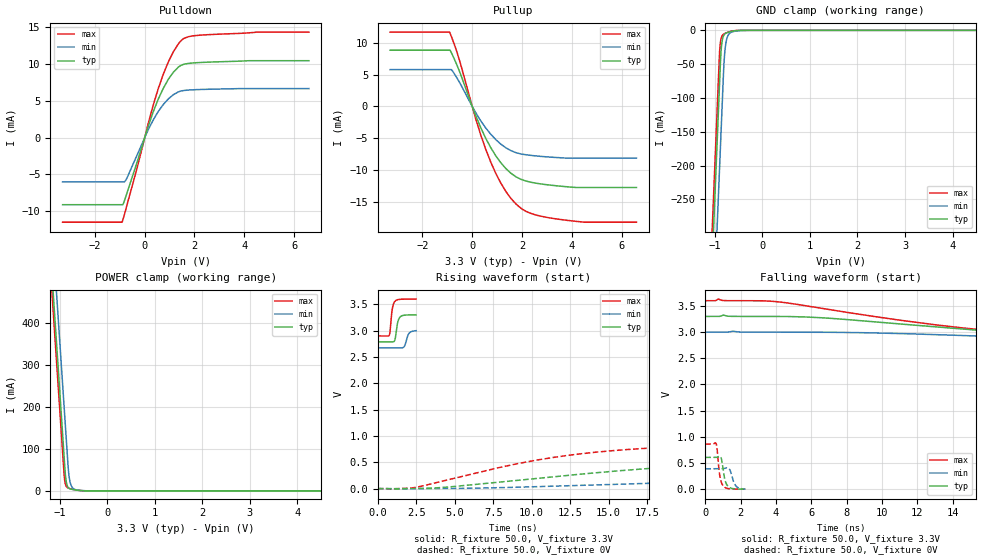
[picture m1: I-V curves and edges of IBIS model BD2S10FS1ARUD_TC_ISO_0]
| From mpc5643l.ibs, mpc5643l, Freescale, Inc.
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| *** New cell (Generated with 5.14beta1 (Sep 20 2010 13:23:23))
[Model]   BD2S10FS1ARUD_TC_ISO_0
Model_type I/O
Polarity   Non-Inverting
Enable   Active-Low
| CAP_THRESHOLD on pad pad is "CMOS" :
| Rising=10.0% of VDDE1   Falling=90.0% of VDDE1
| C_comp min and max val. don't necessarily correlate with the min and max pvt
| but are the smallest and greatest pad capacitance found.
| var   typ   min   max
C_comp   2.15700pF  2.04013pF  2.29327pF
Vinl = 1.05V | Dummy value overriden by next lines
Vinh = 2.34V | Dummy value overriden by next lines
Vmeas = 1.65V   | Reference voltage for timing measurements
Cref  = 25.0pF   | Timing specification test load capacitance value
Rref  = 1.0MOhm   | Timing specification test load resistance value
Vref  = 1.65V   | Timing specification test load voltage
[Model Spec]
| TIME_THRESHOLD on pin ipp_ind is "CORE" :
| Rising=40.0% of VDD   Falling=60.0% of VDD
Vinl 1.32350V 1.20950V 1.42250V
Vinh 1.90350V 1.72650V 2.05550V
| variable   typ   min   max
[Temperature Range] 25.0 150.0 -40.0
| variable   typ   min   max
[Voltage Range] 3.3V 3.0V 3.6V
| variable   typ   min   max
[POWER Clamp Reference] 3.3V 3.0V 3.6V
| variable   typ   min   max
[GND Clamp Reference] 0V 0V 0V
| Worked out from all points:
|   slope of the pulldown table from 0 to 0.495 V, typ, clamps not added: 103 ohm
|   slope of the pullup table from 0 to 0.495 V, typ, clamps not added: 108 ohm
|   GND clamp passes 1 mA (typ) near -0.61 V on its own axis
|   POWER clamp passes 1 mA (typ) near -0.57 V on its own axis
|   rising waveform, R_fixture 50.0, V_fixture 3.3V: 20-80 % time 176ps typ, 215ps min, 157ps max; typ from 2.79 V to 3.3 V
|   falling waveform, R_fixture 50.0, V_fixture 3.3V: 20-80 % time 12.8ns typ, 19.9ns min, 9.33ns max; typ from 3.3 V to 2.79 V
|   rising waveform, R_fixture 50.0, V_fixture 0V: 20-80 % time 16ns typ, 31.9ns min, 9.41ns max; typ from 0 V to 0.606 V
|   falling waveform, R_fixture 50.0, V_fixture 0V: 20-80 % time 202ps typ, 238ps min, 181ps max; typ from 0.606 V to 0 V
[POWER Clamp]
-3.3V     4.147A     4.265A     4.103A
-1.21V    593.6mA    712.4mA    550.2mA
-1.14V    474.6mA    593.4mA    431.2mA
-1.07V    355.6mA    474.4mA    312.2mA
-1V       236.6mA    355.4mA    193.2mA
-900mV    66.63mA    185.4mA    27.75mA
-870mV    26.01mA    134.4mA    12.15mA
-820mV    7.991mA    51.43mA    6.71mA
-790mV    5.39mA     24.66mA    5.573mA
-740mV    3.621mA    8.522mA    4.182mA
-500mV    402.7uA    702.3uA    321.1uA
6.6V      0A         0A         0A
[GND Clamp]
-3.3V     -4.158A    -4.283A    -4.111A
-1.08V    -384.3mA   -509.2mA   -336.5mA
-910mV    -95.27mA   -220.2mA   -47.53mA
-890mV    -61.27mA   -186.2mA   -22.28mA
-880mV    -44.27mA   -169.2mA   -16.28mA
-860mV    -23.44mA   -135.2mA   -10.07mA
-810mV    -7.304mA   -52.22mA   -5.488mA
-790mV    -5.469mA   -31.98mA   -4.717mA
-760mV    -3.985mA   -16.09mA   -3.79mA
-680mV    -2.058mA   -3.959mA   -1.879mA
-460mV    -100.3uA   -366.4uA   -40.84uA
6.6V      10.86nA    3.471uA    69.11pA
| variable   typ   min   max
[Pullup Reference] 3.3V 3.0V 3.6V
| variable   typ   min   max
[Pulldown Reference] 0V 0V 0V
[Pullup]
-3.3V     8.828mA    5.778mA    11.67mA
-910mV    8.828mA    5.778mA    11.67mA
-830mV    8.358mA    5.778mA    10.89mA
-530mV    5.681mA    3.906mA    7.464mA
340mV     -3.31mA    -2.242mA   -4.446mA
740mV     -6.438mA   -4.34mA    -8.697mA
950mV     -7.768mA   -5.218mA   -10.53mA
1.35V     -9.742mA   -6.484mA   -13.33mA
1.96V     -11.44mA   -7.454mA   -15.99mA
2.57V     -12.05mA   -7.77mA    -17.05mA
3.78V     -12.6mA    -8.107mA   -17.86mA
6.6V      -12.72mA   -8.115mA   -18.17mA
[Pulldown]
-3.3V     -9.096mA   -6.007mA   -11.47mA
-910mV    -9.096mA   -6.007mA   -11.47mA
-860mV    -8.955mA   -6.007mA   -10.95mA
-730mV    -7.701mA   -5.58mA    -9.361mA
-270mV    -2.95mA    -2.093mA   -3.641mA
140mV     1.518mA    1.051mA    1.902mA
540mV     5.179mA    3.516mA    6.592mA
950mV     7.904mA    5.249mA    10.26mA
1.15V     8.857mA    5.814mA    11.62mA
1.53V     9.89mA     6.36mA     13.34mA
2.57V     10.23mA    6.552mA    13.95mA
6.6V      10.42mA    6.642mA    14.3mA
[Ramp]
dV/dt_r 363.82411mV/16.01548ns 233.53819mV/31.8706ns 516.40158mV/9.40995ns
dV/dt_f 307.73137mV/12.83706ns 196.81296mV/19.89569ns 420.29549mV/9.33353ns
R_load = 50.0
| Removed startup time: 0s 0s 0s  .
| Removed end time: 2.485ns.
[Rising Waveform]
R_fixture   = 50.0
V_fixture   = 3.3V
V_fixture_min = 3.0V
V_fixture_max = 3.6V
0s        2.787V     2.672V     2.9V
748ps     2.787V     2.672V     2.915V
801ps     2.787V     2.672V     2.995V
939ps     2.785V     2.672V     3.409V
1.112ns   2.825V     2.672V     3.556V
1.284ns   3.145V     2.672V     3.587V
1.426ns   3.251V     2.671V     3.594V
1.727ns   3.293V     2.701V     3.598V
2.048ns   3.298V     2.955V     3.599V
2.487ns   3.3V       3V         3.6V
| Removed startup time: 0s 0s 0s  .
| Removed end time: 89.5ns.
[Falling Waveform]
R_fixture   = 50.0
V_fixture   = 3.3V
V_fixture_min = 3.0V
V_fixture_max = 3.6V
0s        3.3V       3V         3.6V
750ps     3.299V     3V         3.631V
4.1ns     3.3V       3V         3.579V
7ns       3.266V     2.997V     3.431V
14.65ns   3.057V     2.934V     3.078V
17.75ns   2.98V      2.898V     2.991V
21.4ns    2.905V     2.856V     2.948V
28.2ns    2.837V     2.783V     2.92V
40.4ns    2.803V     2.715V     2.905V
89.6ns    2.787V     2.672V     2.9V
| Removed startup time: 0s 0s 0s  .
| Removed end time: 113.2ns.
[Rising Waveform]
R_fixture   = 50.0
V_fixture   = 0V
V_fixture_min = 0V
V_fixture_max = 0V
0s        18.72nV    2.005uV    15.84nV
900ps     324.5uV    1.89uV     -10.23mV
2.5ns     1.08mV     -197.2uV   26.1mV
8.8ns     148.8mV    24.33mV    457.2mV
12.65ns   260.5mV    56.06mV    642.3mV
16.8ns    364.8mV    93.16mV    754mV
21.8ns    457mV      140mV      815.7mV
32.65ns   557.3mV    231.8mV    852.7mV
53.5ns    599.7mV    333.7mV    860.1mV
113.3ns   606.4mV    389.2mV    860.7mV
| Removed startup time: 0s 0s 0s  .
| Removed end time: 2.268ns.
[Falling Waveform]
R_fixture   = 50.0
V_fixture   = 0V
V_fixture_min = 0V
V_fixture_max = 0V
0s        606.4mV    389.4mV    860.7mV
608ps     606.1mV    389.4mV    871mV
666ps     610.1mV    389.3mV    774.1mV
822ps     629mV      389.1mV    253.4mV
922ps     563mV      388.9mV    118.2mV
1.024ns   333.5mV    391.9mV    57.22mV
1.141ns   142.9mV    401.5mV    27.53mV
1.337ns   38.46mV    392.3mV    8.295mV
1.723ns   4.913mV    64.88mV    1.528mV
2.27ns    119.9uV    64.31uV    142.6uV
